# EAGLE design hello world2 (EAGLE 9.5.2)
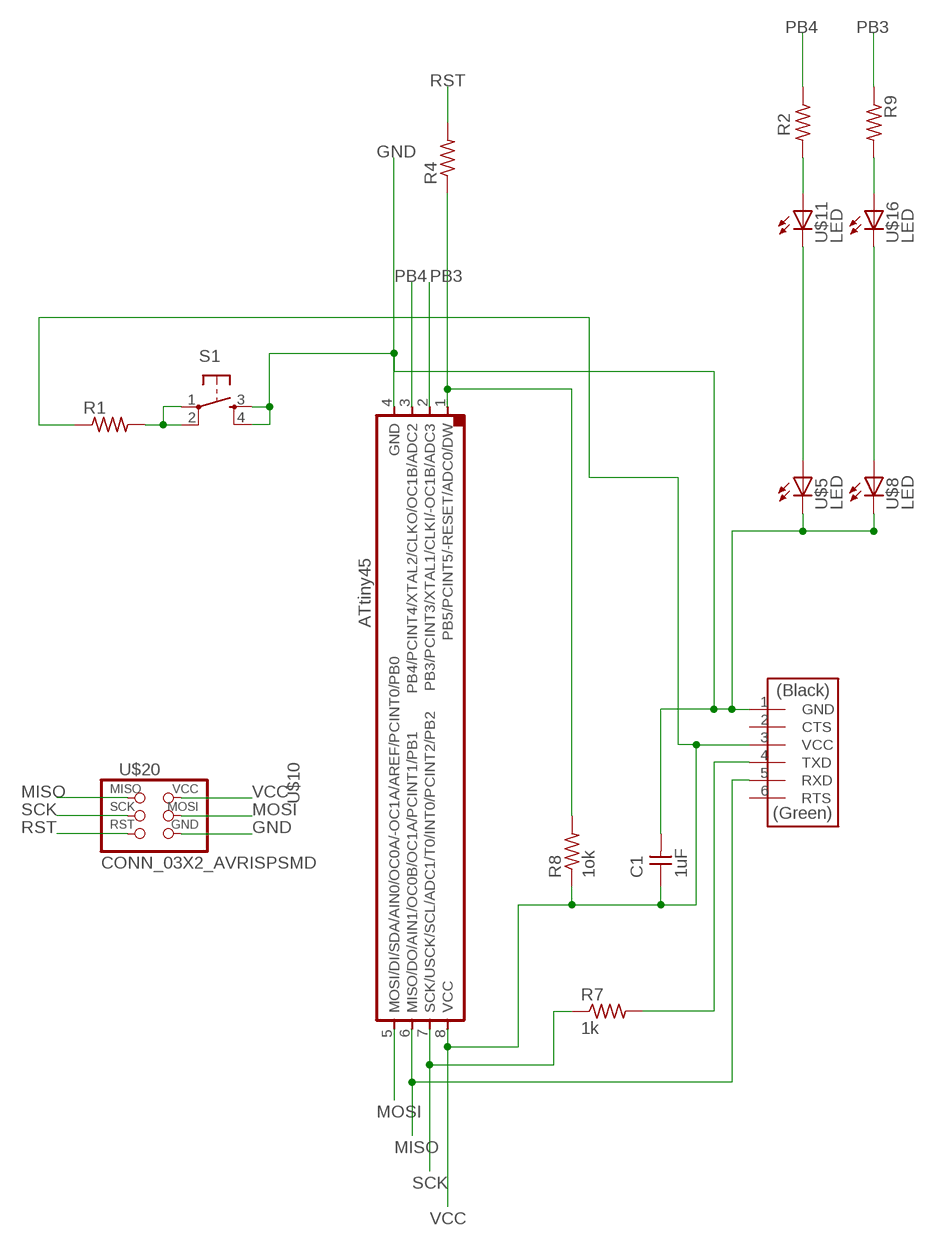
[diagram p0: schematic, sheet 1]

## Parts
C1  1uF  CAP_UNPOLARIZED  [C1206]
R1  R1206  [R1206]
R2  R1206  [R1206]
R4  R1206  [R1206]
R7  1k  R1206  [R1206]
R8  1ok  R1206  [R1206]
R9  R1206  [R1206]
S1  SW_SWITCH_TACTILE_6MM6MM_SWITCH  [6MM_SWITCH]
U$1  CONN_06_FTDI-SMD-HEADER  [1X06SMD]
U$5  LED  [LED1206]
U$8  LED  [LED1206]
U$10  UC_ATTINY45SI  [SOIC8]
U$11  LED  [LED1206]
U$16  LED  [LED1206]
U$20  CONN_03X2_AVRISPSMD  [2X03SMD]

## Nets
GND: C1.2 S1.3(S) S1.4(S1) U$1.1(GND) U$5.2(C) U$8.2(C) U$10.4(GND) U$20.6(GND)
MISO: U$1.5(RXD) U$10.6(MISO/DO/AIN1/OC0B/OC1A/PCINT1/PB1) U$20.1(MISO)
MOSI: U$10.5(MOSI/DI/SDA/AIN0/OC0A/-OC1A/AREF/PCINT0/PB0) U$20.4(MOSI)
N$1: R2.2 U$11.1(A)
N$2: R9.2 U$16.1(A)
N$3: R4.1 R8.2 U$10.1(PB5/PCINT5/-RESET/ADC0/DW)
N$4: U$5.1(A) U$11.2(C)
N$5: U$8.1(A) U$16.2(C)
N$18: R7.2 U$1.4(TXD)
N$24: R1.2 S1.1(P) S1.2(P1)
PB3: R9.1 U$10.2(PB3/PCINT3/XTAL1/CLKI/-OC1B/ADC3)
PB4: R2.1 U$10.3(PB4/PCINT4/XTAL2/CLKO/OC1B/ADC2)
RST: R4.2 U$20.5(RST)
SCK: R7.1 U$10.7(SCK/USCK/SCL/ADC1/T0/INT0/PCINT2/PB2) U$20.3(SCK)
VCC: C1.1 R1.1 R8.1 U$1.3(VCC) U$10.8(VCC) U$20.2(VCC)
Unconnected: U$1.2(CTS) U$1.6(RTS)

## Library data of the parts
C1 = eagle_fab:CAP_UNPOLARIZED
R1 R2 R4 R7-R9 = eagle_fab:R: Resistor (US Symbol)
S1 = eagle_fab:SW_SWITCH_TACTILE_6MM: OMRON SWITCH
U$1 = eagle_fab:CONN_06_FTDI-SMD-HEADER
U$5 U$8 U$11 U$16 = eagle_fab:LED: LED
U$10 = eagle_fab:UC_ATTINY45
U$20 = eagle_fab:CONN_03X2_AVRISP

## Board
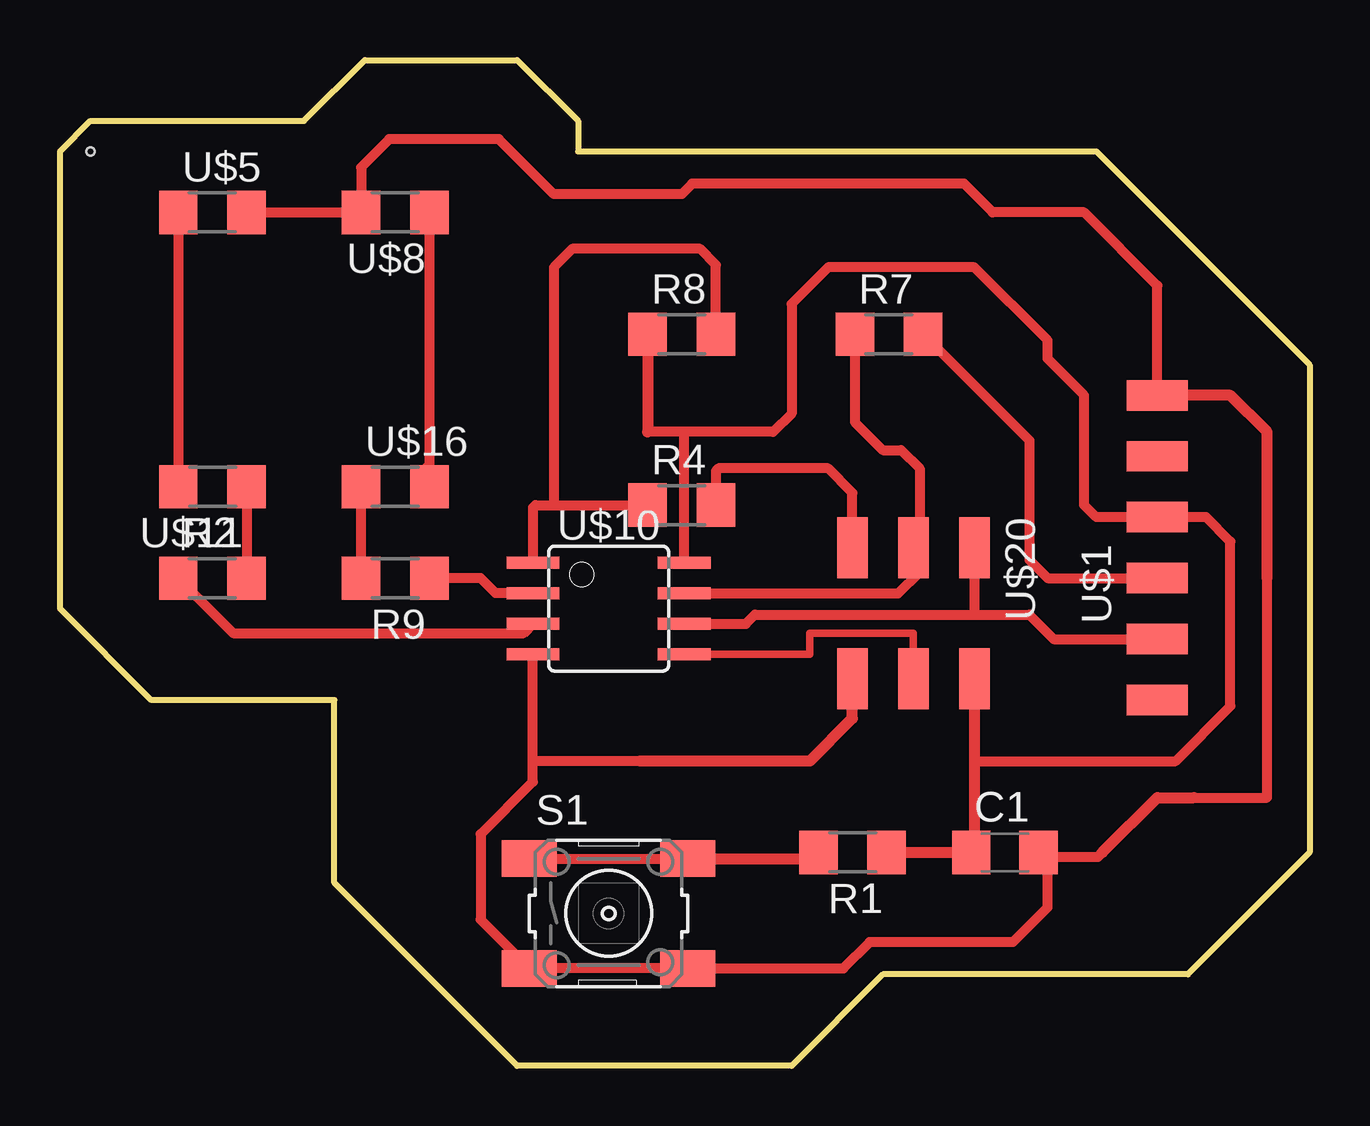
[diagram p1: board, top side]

Size 52.07 x 41.91 mm. Coordinates in mm from the lower left corner, seen from the top.
Outline: 21.59,38.1 43.18,38.1 52.07,29.21 52.07,8.89 46.99,3.81 34.29,3.81 30.48,0 19.05,0 11.43,7.62 11.43,15.24 3.81,15.24 0,19.05 0,38.1 1.27,39.37 10.16,39.37 12.7,41.91 19.05,41.91 21.59,39.37 21.59,38.1
Copper layers (1*16): Top 0.035mm / dielectric 1.5mm / Bottom 0.035mm
Design rules "default *": minimum track width 6mil, minimum drill 0.35mm, track to track 10mil, track to pad 6mil, pad to pad 6mil, via to via 6mil, smd to smd 6mil, copper to edge 40mil, drill to drill 6mil, minimum pad ring 10mil, minimum via ring 8mil, stop-mask expansion 4mil, vias tented up to drill 0mil, thermal gap 10mil
Holes 0.35 mm at 1.27,38.1

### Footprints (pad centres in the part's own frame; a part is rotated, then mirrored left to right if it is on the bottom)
C1206 = smd 1.6 x 1.8: 1 -1.4,0; 2 1.4,0
R1206 = smd 1.6 x 1.803: 1 -1.422,0; 2 1.422,0
6MM_SWITCH = smd 2.286 x 1.524: 1 -3.302,2.286; 2 3.302,2.286; 3 -3.302,-2.286; 4 3.302,-2.286
1X06SMD = smd 2.54 x 1.27: 1 0,6.35; 2 0,3.81; 3 0,1.27; 4 0,-1.27; 5 0,-3.81; 6 0,-6.35
LED1206 = smd 1.6 x 1.803: 1 -1.422,0; 2 1.422,0
SOIC8 = smd 0.5 x 2.2: 1 -1.905,-3.154; 2 -0.645,-3.154; 3 0.625,-3.154; 4 1.895,-3.154; 5 1.905,3.154; 6 0.635,3.154; 7 -0.635,3.154; 8 -1.905,3.154
2X03SMD = smd 2.54 x 1.27: 1 -2.54,2.54; 2 2.92,2.54; 3 -2.54,0; 4 2.92,0; 5 -2.54,-2.54; 6 2.92,-2.54

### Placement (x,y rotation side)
C1  39.37,8.89 0 top
R1  33.02,8.89 180 top
R2  6.35,20.32 0 top
R4  25.91,23.37 0 top
R7  34.54,30.48 0 top
R8  25.91,30.48 0 top
R9  13.97,20.32 180 top
S1  22.86,6.35 0 top
U$1  45.72,21.59 0 top
U$5  6.35,35.56 0 top
U$8  13.97,35.56 180 top
U$10  22.86,19.05 270 top
U$11  6.35,24.13 180 top
U$16  13.97,24.13 0 top
U$20  35.56,19.05 270 top

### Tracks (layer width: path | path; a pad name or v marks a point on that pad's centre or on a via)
GND
  Top 0.254: 19.69,17.16 U$10.4
  Top 0.406: U$5.2 U$8.2 12.55,37.44 13.72,38.61 18.29,38.61 20.57,36.32 25.91,36.32 26.34,36.75 37.67,36.75 38.86,35.56 42.67,35.56 45.72,32.51 U$1.1 | 47.24,11.18 50.29,11.18 50.29,20.32 | 40.96,8.7 41.15,8.51 41.15,6.6 39.7,5.16 33.73,5.16 32.64,4.06 S1.4 S1.3 17.53,6.1 17.53,9.65 19.71,11.83 19.71,12.7 | 40.96,8.7 C1.2 | 43.43,8.89 43.24,8.7 40.96,8.7 | 19.71,12.7 U$10.4 19.69,17.16 | 24.16,12.7 19.71,12.7
  Top 0.457: 24.16,12.7 31.24,12.7 33.02,14.48 U$20.6 | 47.24,11.18 45.72,11.18 43.43,8.89 | 50.29,20.32 50.29,26.42 48.77,27.94 U$1.1
MISO
  Top 0.406: U$10.6 28.58,18.41 28.96,18.8 38.1,18.8 | 38.1,18.8 40.39,18.8 41.4,17.78 U$1.5 | U$20.1 38.1,18.8
MOSI
  Top 0.305: U$20.4 35.56,18.03 31.24,18.03 31.24,17.14 U$10.5
N$1
  Top 0.406: U$11.1 R2.2
N$2
  Top 0.406: R9.2 U$16.1
N$3
  Top 0.406: 20.57,23.37 19.81,23.37 19.71,23.26 U$10.1 | 20.57,23.37 R4.1 | R8.2 27.33,33.38 26.67,34.04 21.34,34.04 20.57,33.27 20.57,23.37
N$4
  Top 0.406: U$5.1 U$11.2
N$5
  Top 0.406: U$8.1 15.39,25.04 15.24,24.89 15.24,24.28 U$16.2
N$18
  Top 0.406: R7.2 40.39,26.06 40.39,21.08 41.15,20.32 U$1.4
N$24
  Top 0.406: S1.1 S1.2
  Top 0.457: S1.2 31.34,8.64 R1.2
PB3
  Top 0.406: U$10.2 18.15,19.7 17.53,20.32 R9.1
PB4
  Top 0.406: R2.1 7.21,18.03 19.31,18.03 U$10.3
RST
  Top 0.406: U$20.5 33.02,23.88 32,24.89 27.43,24.89 27.33,24.79 R4.2
SCK
  Top 0.406: R7.1 33.12,26.82 34.29,25.65 35.05,25.65 35.81,24.89 35.81,21.84 U$20.3 35.81,21.34 35.81,20.57 34.92,19.69 U$10.7
VCC
  Top 0.254: 38.03,8.95 C1.1
  Top 0.406: 38.1,12.7 46.48,12.7 48.77,14.99 48.77,21.84 47.75,22.86 U$1.3 43.18,22.86 42.67,23.37 42.67,27.94 41.15,29.46 41.15,30.23 38.1,33.27 32,33.27 30.48,31.75 30.48,27.18 29.72,26.42 25.91,26.42 | 25.91,26.42 24.49,26.42 | U$10.8 26.01,26.31 25.91,26.42
  Top 0.457: R1.1 C1.1 | U$20.2 38.1,12.7 38.1,9.02 38.03,8.95 | R8.1 24.49,26.42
